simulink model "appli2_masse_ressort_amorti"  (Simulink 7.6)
settings: Solver=ode15s  StartTime=0.0  StopTime=1.0  RelTol=1e-3
InitFcn:
  | f=10;
  | m=1;
  | k=1000;
StopFcn:
  | close all
  | load pos_vit.mat
  | plotyy(pv(1,:),pv(2,:),pv(1,:),pv(3,:))
  | gtext('Vitesse en ms/s')
  | gtext('Position en m')
  | title('Vitesse et position de la masse')
  | xlabel('temps')
  | grid
  | hold on
  | plot(pv(1,:),pv(4,:))
  | gtext('enveloppe')
libraries: fl_lib x7, nesl_utility x3

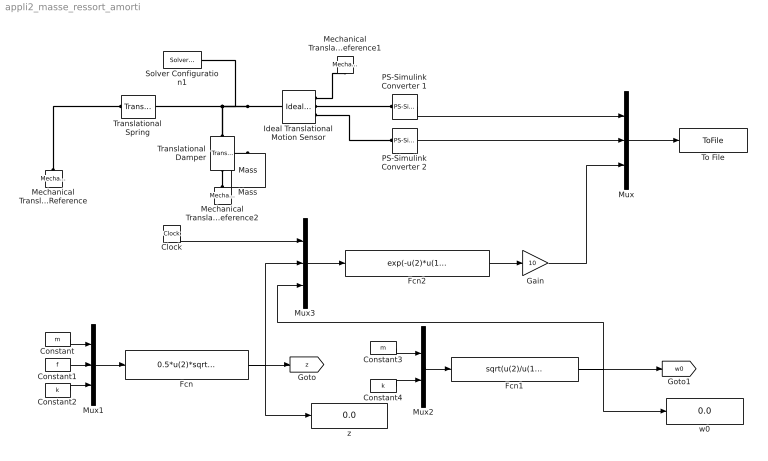
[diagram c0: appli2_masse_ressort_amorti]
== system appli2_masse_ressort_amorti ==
  Clock : Clock
  Constant : Constant  Value=m
  Constant1 : Constant  Value=f
  Constant2 : Constant  Value=k
  Constant3 : Constant  Value=m
  Constant4 : Constant  Value=k
  Fcn : Fcn  Expr=0.5*u(2)*sqrt(1/(u(3)*u(1)))
  Fcn1 : Fcn  Expr=sqrt(u(2)/u(1))
  Fcn2 : Fcn  Expr=exp(-u(2)*u(1)*u(3))
  Gain : Gain  Gain=10
  Ideal Translational Motion Sensor : fl_lib/Mechanical/Mechanical Sensors/Ideal Translational Motion Sensor  DialogController=NetworkEngine.DynNeDlgSource  SystemSampleTime=-1  offset=0 m  v_Log=off  f_Log=off  x_Log=off  LocalVarNames=|v|f|x  LocalVarDescs=|v|f|x  LocalVarLogging=[0 0 0]
  Mass : fl_lib/Mechanical/Translational Elements/Mass  DialogController=NetworkEngine.DynNeDlgSource  SystemSampleTime=-1  mass=m kg  initial_velocity=10 m/s  f_Log=off  LocalVarNames=|f  LocalVarDescs=|f  LocalVarLogging=0
  Mechanical Translational Reference : fl_lib/Mechanical/Translational Elements/Mechanical Translational Reference  DialogController=NetworkEngine.DynNeDlgSource  SystemSampleTime=-1  f_Log=off  LocalVarNames=|f  LocalVarDescs=|f  LocalVarLogging=0
  Mechanical Translational Reference1 : fl_lib/Mechanical/Translational Elements/Mechanical Translational Reference  DialogController=NetworkEngine.DynNeDlgSource  SystemSampleTime=-1  f_Log=off  LocalVarNames=|f  LocalVarDescs=|f  LocalVarLogging=0
  Mechanical Translational Reference2 : fl_lib/Mechanical/Translational Elements/Mechanical Translational Reference  DialogController=NetworkEngine.DynNeDlgSource  SystemSampleTime=-1  f_Log=off  LocalVarNames=|f  LocalVarDescs=|f  LocalVarLogging=0
  Mux : Mux  Inputs=3
  Mux1 : Mux  Inputs=3
  Mux2 : Mux  Inputs=2
  Mux3 : Mux  Inputs=3
  PS-Simulink Converter 1 : nesl_utility/PS-Simulink Converter  DialogController=NetworkEngine.DynNeUtilDlgSource  SystemSampleTime=-1  PhysicalDomain=network_engine_domain  LeftPortType=input  RightPortType=output  SubClassName=ps_output  Unit=1  AffineConversion=off
  PS-Simulink Converter 2 : nesl_utility/PS-Simulink Converter  DialogController=NetworkEngine.DynNeUtilDlgSource  SystemSampleTime=-1  PhysicalDomain=network_engine_domain  LeftPortType=input  RightPortType=output  SubClassName=ps_output  Unit=1  AffineConversion=off
  Solver Configuration1 : nesl_utility/Solver Configuration  DialogController=NetworkEngine.DynNeUtilDlgSource  SystemSampleTime=-1  PhysicalDomain=network_engine_domain  LeftPortType=input  RightPortType=generic  SubClassName=solver  Accelerate=off  Profile=off  ResidualTolerance=1e-9  MaxNonlinIter=12  MaxModeIter=2  DoFixedCost=off  UseLocalSampling=off  DoDC=off  LinearAlgebra=Sparse  LocalSolverSampleTime=.001  LocalSolverChoice=NE_BACKWARD_EULER_ADVANCER  UseLocalSolver=off
  To File : ToFile  Filename=pos_vit.mat  MatrixName=pv
  Translational Damper : fl_lib/Mechanical/Translational Elements/Translational Damper  DialogController=NetworkEngine.DynNeDlgSource  SystemSampleTime=-1  D=f N/(m/s)  f_Log=off  v_Log=off  LocalVarNames=|f|v  LocalVarDescs=|f|v  LocalVarLogging=[0 0]
  Translational Spring : fl_lib/Mechanical/Translational Elements/Translational Spring  DialogController=NetworkEngine.DynNeDlgSource  SystemSampleTime=-1  spr_rate=k N/m  init_def=0 m  f_Log=off  v_Log=off  x_Log=off  LocalVarNames=|f|v|x  LocalVarDescs=|f|v|x  LocalVarLogging=[0 0 0]
  w0 : Display
  z : Display
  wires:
  PS-Simulink Converter 1/1 -> Mux/1
  PS-Simulink Converter 2/1 -> Mux/2
  Mux/1 -> To File/1
  Fcn/1 -> [z], z/1, Mux3/2
  Constant/1 -> Mux1/1
  Constant1/1 -> Mux1/2
  Constant2/1 -> Mux1/3
  Mux1/1 -> Fcn/1
  Mux2/1 -> Fcn1/1
  Constant4/1 -> Mux2/2
  Constant3/1 -> Mux2/1
  Fcn1/1 -> w0/1, [w0], Mux3/3
  Fcn2/1 -> Gain/1
  Clock/1 -> Mux3/1
  Mux3/1 -> Fcn2/1
  Gain/1 -> Mux/3
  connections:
  Ideal Translational Motion Sensor/LConn1 -- Mass/LConn1 -- Solver Configuration1/RConn1 -- Translational Damper/LConn1 -- Translational Spring/RConn1
  Mechanical Translational Reference/LConn1 -- Translational Spring/LConn1
  Ideal Translational Motion Sensor/RConn1 -- Mechanical Translational Reference1/LConn1
  Ideal Translational Motion Sensor/RConn2 -- PS-Simulink Converter 1/LConn1
  Ideal Translational Motion Sensor/RConn3 -- PS-Simulink Converter 2/LConn1
  Translational Damper/RConn1 -- Mechanical Translational Reference2/LConn1
